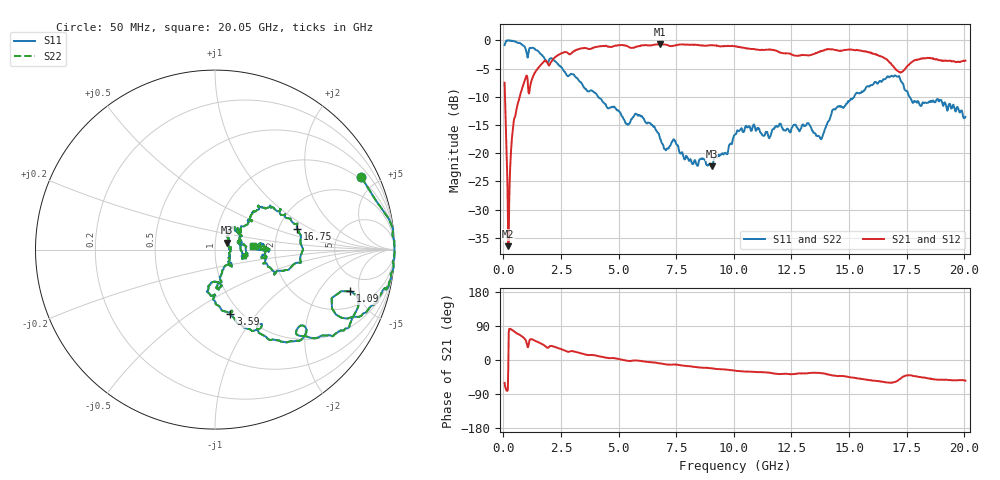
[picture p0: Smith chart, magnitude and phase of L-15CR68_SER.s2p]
! P/N: L-15CR68JE
! Measured by Marlon
! Oct. 13, 2003
! Measure with Series-through-Fixture
#	mhz	s	ma	r	50
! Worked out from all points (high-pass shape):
!   1001 points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, 50 MHz to 20.05 GHz, reference 50 ohm
!   highest |S21| = -0.68 dB at 6.79 GHz (marker M1); lowest = -36.5 dB at 210 MHz (marker M2)
!   |S21| within 3 dB of the highest: 2.091 GHz to 16.71 GHz (14.62 GHz wide, 156 % of centre); 17.78 GHz to 19.42 GHz (1.638 GHz wide, 8.81 % of centre)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
!   lowest |S11| = -22.3 dB at 9.03 GHz (marker M3), VSWR 1.17, Z = 56.9 + j4.43 ohm
!   |S11| at or under -10 dB: 4.108 GHz to 15.22 GHz (11.11 GHz wide, 115 % of centre); 17.63 GHz to end of sweep
!   |S22| runs from -22.3 to 0.0 dB; largest |S21 - S12| = 0
!   S11 on the Smith chart (normalised r, x): 50 MHz: 0.88, +4.11; 1.09 GHz: 3.30, -4.07; 3.59 GHz: 0.90, -0.74; 16.75 GHz: 2.52, +0.76; 20.05 GHz: 1.53, +0.07
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50  0.9097 26.2  0.4218 -60.5  0.4218 -60.5  0.9097 26.2
210  1 -0.0  0.015 -17.3  0.015 -17.3  1 -0.0
290  0.9975 -4.6  0.07353 82.6  0.07353 82.6  0.9975 -4.6
390  0.9905 -10.1  0.1512 78.3  0.1512 78.3  0.9905 -10.1
530  0.9779 -12.6  0.2242 72.4  0.2242 72.4  0.9779 -12.6
930  0.8682 -25.5  0.445 55.4  0.445 55.4  0.8682 -25.5
1090  0.7893 -17.1  0.3439 39.9  0.3439 39.9  0.7893 -17.1
2210  0.6604 -50.7  0.7023 35.0  0.7023 35.0  0.6604 -50.7
3390  0.4181 -73.6  0.8504 17.4  0.8504 17.4  0.4181 -73.6
3590  0.3681 -76.6  0.8546 13.9  0.8546 13.9  0.3681 -76.6
6730  0.1503 -78.0  0.9211 -8.6  0.9211 -8.6  0.1503 -78.0
6790  0.1371 -73.7  0.9252 -8.9  0.9252 -8.9  0.1371 -73.7
9030  0.07632 30.5  0.9083 -22.0  0.9083 -22.0  0.07632 30.5
10050  0.1463 55.1  0.8903 -27.9  0.8903 -27.9  0.1463 55.1
13390  0.1596 -8.3  0.7487 -33.8  0.7487 -33.8  0.1596 -8.3
13810  0.1349 19.5  0.8053 -34.9  0.8053 -34.9  0.1349 19.5
14350  0.2455 41.9  0.8253 -40.9  0.8253 -40.9  0.2455 41.9
15390  0.3417 45.5  0.8189 -48.9  0.8189 -48.9  0.3417 45.5
16730  0.4729 15.6  0.6512 -59.8  0.6512 -59.8  0.4729 15.6
16750  0.4717 14.3  0.6402 -60.1  0.6402 -60.1  0.4717 14.3
17430  0.3632 -20.0  0.5589 -41.8  0.5589 -41.8  0.3632 -20.0
20050  0.2101 5.8  0.6617 -54.4  0.6617 -54.4  0.2101 5.8
